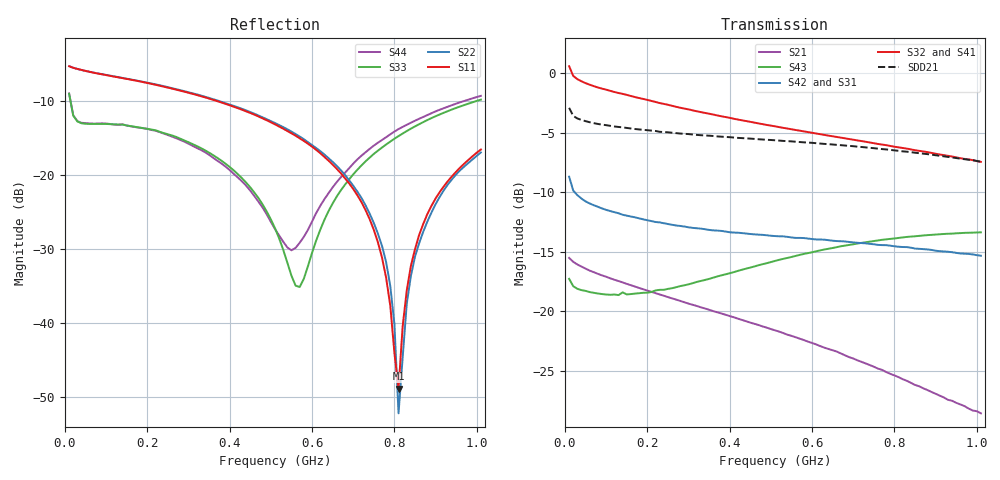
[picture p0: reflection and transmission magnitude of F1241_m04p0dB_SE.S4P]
! Integrated Device Technology
! Corporate Headquarters
! 6024 Silver Creek Valley Road
! San Jose, CA 95138  USA
! Phone:  1-408-284-8200
! Toll Free:  1-800-223-1366
! Webpage:  http://www.idt.com/
! Timing and RF Division
! 515 Groton Road, Suite 102
! Westford, MA 01886-6024
! Device:  F1241
! Description: Dual Intermediate Frequency Digital Variable Gain Amplifier
! Frequency:  10.0 -  500.00 MHz
! Package:  5x5 mm QFN Plastic Package: 32 pin
! Ports:  8 RF, 20 DC
!  Pin  1  = GA3  Pin 17  = RF OUT_B+
!  Pin  2  = GA4  Pin 18  = RF OUT_B-
!  Pin  3  = GA5  Pin 19  = STBY_B
!  Pin  4  = ISET_A  Pin 20  = Ground
!  Pin  5  = ISET_B  Pin 21  = Ground
!  Pin  6  = GB5  Pin 22  = STB_A
!  Pin  7  = GB4  Pin 23  = RF OUT_A-  = Port 4
!  Pin  8  = GB3  Pin 24  = RF OUT_A+  = Port 3
!  Pin  9  = GB2  Pin 25  = NO CONNECT
!  Pin 10  = GB1  Pin 26  = NO CONNECT
!  Pin 11  = RF IN_B+  Pin 27  = VCC
!  Pin 12  = RF IN_B-  Pin 28  = Ground
!  Pin 13  = Ground  Pin 29  = RF IN_A-  = Port 2
!  Pin 14  = VCC  Pin 30  = RF IN_A+  = Port 1
!  Pin 15  = NO CONNECT  Pin 31  = GA1
!  Pin 16  = NO CONNECT  Pin 32  = GA2
! State:  24
! Gain State:  -4.0 dB
! Voltages:  Vcc = +5.00 Volts  Icc approximately 160.0 mA or 80 mA per channel.
! Data:  The device was measured on a custom evaluation board which has
!  individual transmission lines to the RF pins.  Data was collected
!  using a calibrated network analyzer.  The evaluation board was
!  de-embedded using a port reference technique.
!  The reference plane is the edge of the package pin.
!  Only Channel A was measured.
!  This data is in single-ended operation.  If your needs are balanced
!  or differential S-parameters then this file needs to be used a
!  linear simulator.
! Misc:  Lot Code  160028MY
!  Action Tracker AT004
! Date Measured:  2014-08-14
! Date:  2014-08-28  MJV
! Note:
!  Integrated Device Technology supplies this data as a sample of measured
!  data at the package pin for this product.  Your particular data for this
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# Hz S dB R 50
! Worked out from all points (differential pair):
!   101 points, 10 MHz to 1.01 GHz, reference 50 ohm
!   strongest paths, dB at 10 MHz, 260 MHz, 510 MHz, 760 MHz, 1.01 GHz:
!     S32: 0.6, -2.8, -4.5, -6.0, -7.5
!     S41: 0.6, -2.8, -4.6, -6.2, -7.7
!     S42: -8.7, -12.7, -13.7, -14.4, -15.3
!     S31: -8.7, -12.8, -13.8, -14.6, -15.5
!     S43: -17.3, -18.1, -15.8, -14.1, -13.4
!     S21: -15.5, -18.9, -21.6, -24.8, -28.6
!   taken as a pair (ports 2,1 in; 3,4 out), SDD21 dB: -2.9, -5.0, -5.6, -6.3, -7.4
!   lowest |S11| = -48.8 dB at 810 MHz (marker M1), VSWR 1.01, Z = 49.7 - j0.111 ohm
!   |S11| at or under -10 dB: 367.9 MHz to end of sweep
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1e7  -5.32 -6.3  -15.51 -10.8  -34.40 -2.9  -24.31 7.4
     -15.53 -10.8  -5.31 -6.2  -24.32 7.1  -34.42 -2.9
     -8.70 156.7  0.58 167.7  -9.04 -41.8  -17.32 179.4
     0.62 167.8  -8.70 156.8  -17.28 179.4  -8.99 -41.6
5.6e8  -14.70 -34.7  -22.15 -45.0  -34.87 5.9  -25.54 -26.0
       -22.18 -45.3  -14.47 -31.4  -25.24 -25.9  -34.79 3.7
       -13.93 41.4  -4.78 104.9  -34.93 42.2  -15.48 83.6
       -4.90 103.5  -13.85 40.3  -15.36 83.4  -29.83 66.0
6.6e8  -19.16 -39.0  -23.34 -47.8  -34.08 4.8  -25.52 -31.0
       -23.39 -48.3  -18.76 -35.0  -25.09 -31.0  -33.99 2.3
       -14.23 26.0  -5.37 95.2  -22.89 127.0  -14.76 70.4
       -5.53 93.7  -14.11 24.4  -14.62 70.2  -20.95 118.6
7.8e8  -33.90 -51.8  -24.94 -49.6  -33.02 1.5  -25.57 -37.3
       -25.11 -49.6  -31.78 -37.4  -25.01 -37.7  -33.07 -0.9
       -14.61 9.5  -6.06 83.8  -15.87 129.4  -14.13 55.6
       -6.28 82.4  -14.45 7.2  -13.97 55.4  -14.89 123.6
8.1e8  -48.84 -162.0  -25.40 -49.3  -32.84 0.7  -25.59 -38.9
       -25.54 -49.5  -52.15 -5.0  -25.00 -39.5  -32.78 -1.6
       -14.74 5.8  -6.24 81.1  -14.75 128.7  -14.00 52.1
       -6.47 79.7  -14.59 3.3  -13.85 51.9  -13.80 123.6
8.6e8  -28.09 138.5  -26.16 -48.9  -32.45 -1.4  -25.63 -41.5
       -26.30 -48.9  -29.21 137.6  -24.99 -42.3  -32.40 -3.9
       -14.89 -0.4  -6.53 76.4  -13.14 127.3  -13.83 46.4
       -6.78 75.1  -14.76 -3.0  -13.67 46.2  -12.41 123.1
1.01e9  -16.56 130.7  -28.35 -42.4  -31.51 -8.2  -25.89 -49.5
        -28.58 -42.0  -16.95 131.5  -25.07 -50.7  -31.43 -11.1
        -15.47 -16.7  -7.46 63.1  -9.83 123.0  -13.54 30.5
        -7.75 62.2  -15.34 -20.1  -13.38 30.5  -9.32 119.2
